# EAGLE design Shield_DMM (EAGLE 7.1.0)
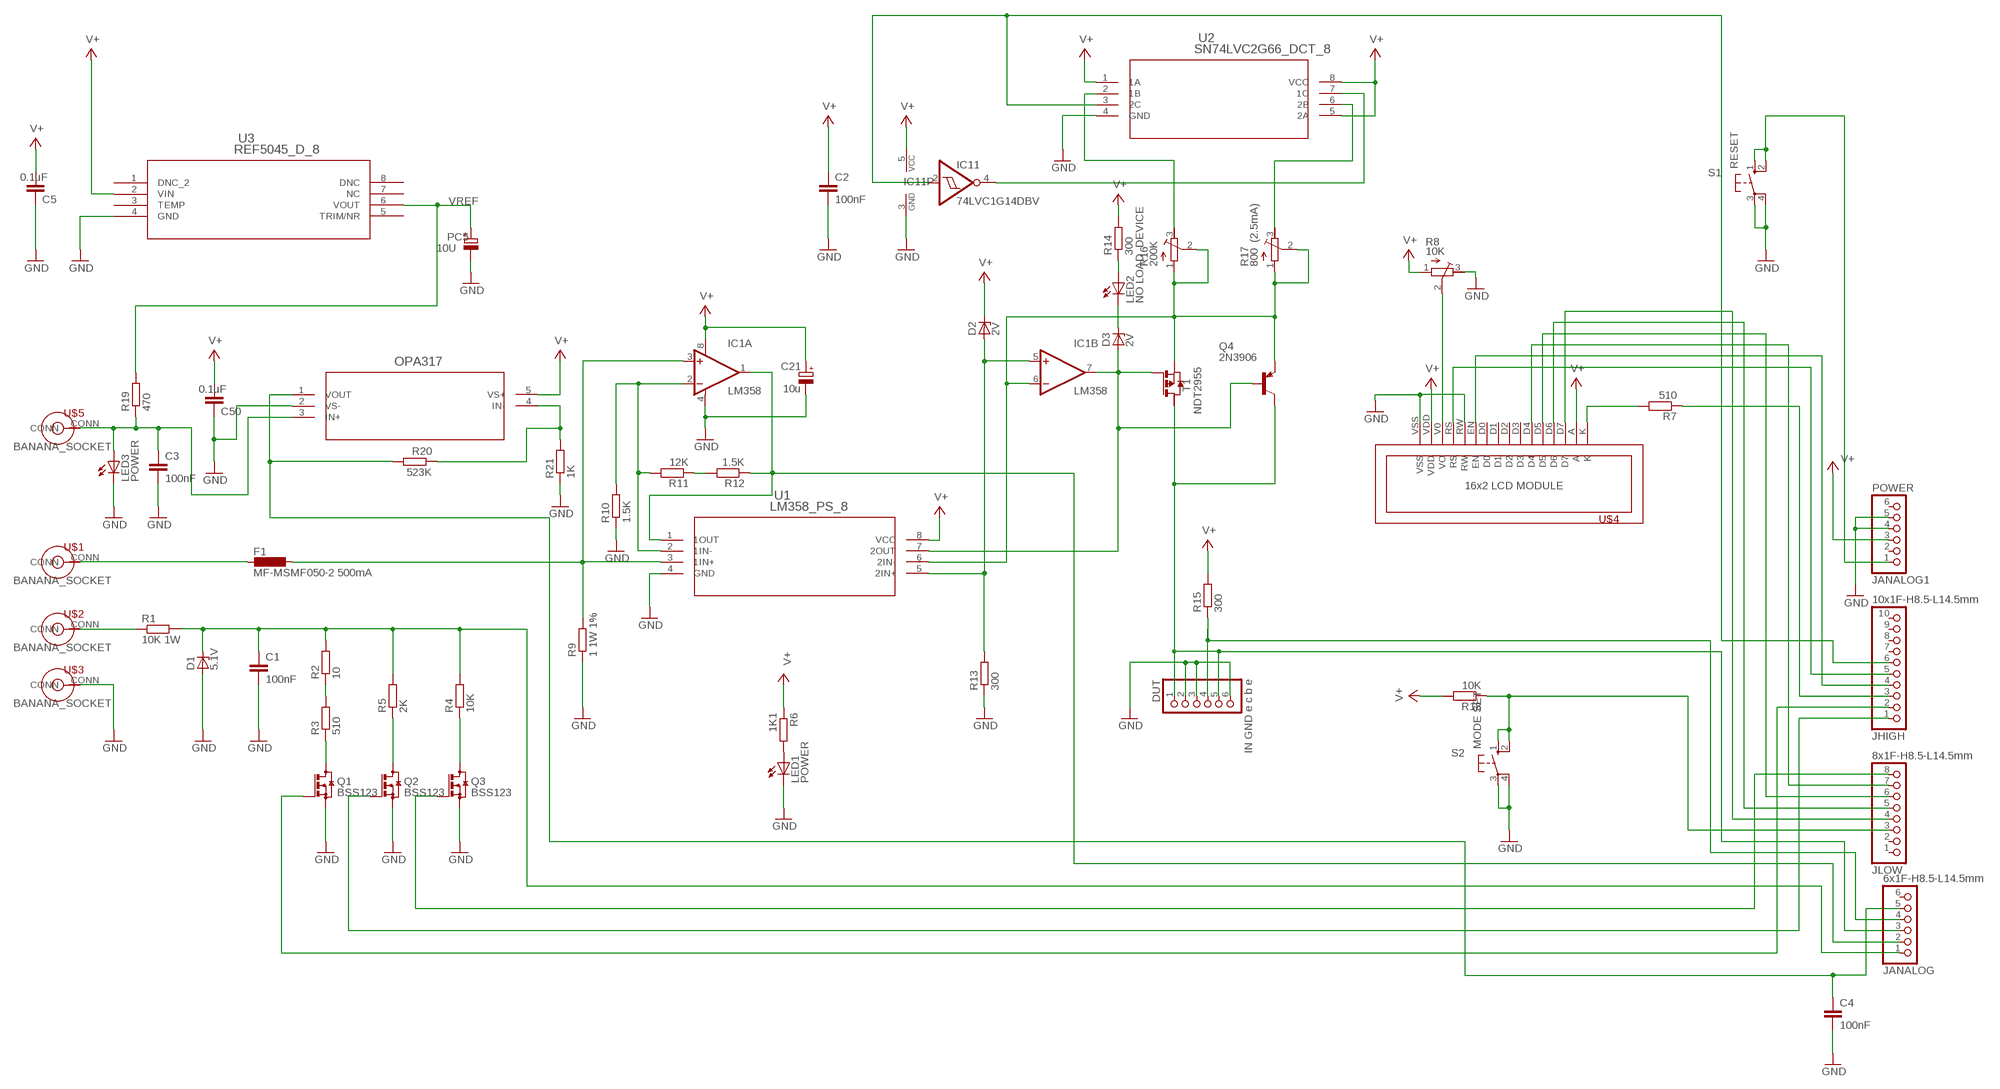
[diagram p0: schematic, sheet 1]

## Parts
C1  100nF  C-EUC0805  [C0805]
C2  100nF  C-EUC0805  [C0805]
C3  100nF  C-EUC0805  [C0805]
C4  100nF  C-EUC0805  [C0805]
C5  0.1uF  C-EUC0805  [C0805]
C21  10u  CPOL-EU085CS-1AR  [085CS_1AR]
C50  0.1uF  C-EUC0805  [C0805]
D1  5.1V  BZV10  [DO34Z7]
D2  2V  BZV10  [DO34Z7]
D3  2V  BZV10  [DO34Z7]
DUT  IN GND e c b e  PINHD-1X6  [1X06]
F1  MF-MSMF050-2 500mA  L-EUL1812  [L1812]
IC1  LM358  OPA2340U  [SO08]
IC11  74LVC1G14DBV  [SOT23-5]
JANALOG  6x1F-H8.5-L14.5mm  PINHD-1X6  [1X06]
JANALOG1  POWER  PINHD-1X6  [1X06]
JHIGH  10x1F-H8.5-L14.5mm  PINHD-1X10  [1X10]
JLOW  8x1F-H8.5-L14.5mm  PINHD-1X8  [1X08]
LED1  POWER  LEDCHIPLED_0805  [CHIPLED_0805]
LED2  NO LOAD DEVICE  LEDCHIPLED_0805  [CHIPLED_0805]
LED3  POWER  LEDCHIPLED_0805  [CHIPLED_0805]
OPA317  THS4281_DBV_5  [DBV5]
PC5  10U  CPOL-EUCT7343  [CT7343]
Q1  BSS123  [SOT23]
Q2  BSS123  [SOT23]
Q3  BSS123  [SOT23]
Q4  2N3906  [TO92]
R1  10K 1W  R-EU_0207/10  [0207/10]
R2  10  R-EU_R0805  [R0805]
R3  510  R-EU_R0805  [R0805]
R4  10K  R-EU_R0805  [R0805]
R5  2K  R-EU_R0805  [R0805]
R6  1K1  R-EU_R0805  [R0805]
R7  510  R-EU_R0805  [R0805]
R8  10K  R-TRIMM64W  [RTRIM64W]
R9  1 1W 1%  R-EU_0207/10  [0207/10]
R10  1.5K  R-EU_R0805  [R0805]
R11  12K  R-EU_R0805  [R0805]
R12  1.5K  R-EU_R0805  [R0805]
R13  300  R-EU_R0805  [R0805]
R14  300  R-EU_R0805  [R0805]
R15  300  R-EU_R0805  [R0805]
R16  200K  R-TRIMM64W  [RTRIM64W]
R17  800 (2.5mA)  R-TRIMM64W  [RTRIM64W]
R18  10K  R-EU_R0805  [R0805]
R19  470  R-EU_R0805  [R0805]
R20  523K  R-EU_R0603  [R0603]
R21  1K  R-EU_R0805  [R0805]
S1  RESET  10-XX  [B3F-10XX]
S2  MODE SET  10-XX  [B3F-10XX]
T1  NDT2955  PMOSSOT223  [SOT223]
U1  LM358_PS_8  [PS8]
U2  SN74LVC2G66_DCT_8  [DCT8]
U3  REF5045_D_8  REF5050_D_8  [D8]
U$1  BANANA_CONN  [BANANA_CONN]
U$2  BANANA_CONN  [BANANA_CONN]
U$3  Common  BANANA_CONN  [BANANA_CONN]
U$4  1602_LCM  [1602_LCM]
U$5  BANANA_CONN  [BANANA_CONN]

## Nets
GND: C1.2 C2.2 C3.2 C4.2 C5.2 C21.- C50.2 D1.A DUT.2 DUT.3 DUT.6 IC1.4(A:V-) IC11.3(GND) JANALOG1.4 JANALOG1.5 LED1.C LED3.C OPA317.2(VS-) PC5.- Q1.2(S) Q2.2(S) Q3.2(S) R8.3(E) R9.1 R10.1 R13.1 R21.1 S1.3(P) S1.4(P1) S2.3(P) S2.4(P1) U1.4(GND) U2.4(GND) U3.4(GND) U$3.CONN U$4.RW U$4.VSS
N$1: R1.1 U$2.CONN
N$2: C1.1 D1.C JANALOG.1 R1.2 R2.2 R4.2 R5.2
N$3: JHIGH.1 Q2.1(G)
N$4: Q3.3(D) R4.1
N$5: R2.1 R3.2
N$6: Q1.3(D) R3.1
N$7: JHIGH.2 Q1.1(G)
N$8: JLOW.8 Q3.1(G)
N$9: Q2.3(D) R5.1
N$10: LED1.A R6.2
N$11: R7.2 U$4.K
N$12: JHIGH.3 R7.1
N$13: R8.2(S) U$4.V0(VO)
N$14: JHIGH.4 U$4.EN
N$15: JHIGH.5 U$4.RS
N$16: JLOW.7 U$4.D4
N$17: JLOW.6 U$4.D5
N$18: JLOW.4 U$4.D7
N$19: JLOW.3 R18.1 S2.1(S) S2.2(S1)
N$20: F1.2 U$1.CONN
N$21: F1.1 IC1.3(A:+IN) R9.2 U1.3(1IN+)
N$22: IC1.2(A:-IN) R10.2 R11.2 U1.2(1IN-)
N$23: D2.A IC1.5(B:+IN) R13.2 U1.5(2IN+)
N$24: R11.1 R12.2
N$25: IC1.1(A:OUT) JANALOG.2 R12.1 U1.1(1OUT)
N$26: OPA317.4(IN-) R20.1 R21.2
N$27: IC1.6(B:-IN) Q4.3(E) R16.1(A) R16.2(S) R17.1(A) R17.2(S) T1.3(S) U1.6(2IN-)
N$28: D3.C LED2.C
N$29: LED2.A R14.1
N$30: DUT.1 DUT.5 JANALOG.3 Q4.1(C) T1.2(D)
N$31: JANALOG1.1 S1.1(S) S1.2(S1)
N$32: DUT.4 JANALOG.4 R15.1
N$33: JLOW.5 U$4.D6
N$34: IC11.2(I) JHIGH.6 U2.3(2C)
N$35: R16.3(E) U2.2(1B)
N$36: IC11.4(O) U2.7(1C)
N$38: D3.A IC1.7(B:OUT) Q4.2(B) T1.1(G) U1.7(2OUT)
N$39: R17.3(E) U2.6(2B)
V+: C2.1 C5.1 C21.+ C50.1 D2.C IC1.8(A:V+) IC11.5(VCC) JANALOG1.3 OPA317.5(VS+) R6.1 R8.1(A) R14.2 R15.2 R18.2 U1.8(VCC) U2.1(1A) U2.5(2A) U2.8(VCC) U3.2(VIN) U$4.A U$4.VDD
VR: C3.1 LED3.A OPA317.3(IN+) R19.1 U$5.CONN
VR1: C4.1 JANALOG.5 OPA317.1(VOUT) R20.2
VREF: PC5.+ R19.2 U3.6(VOUT)
Unconnected: JANALOG1.2 JANALOG1.6 JANALOG.6 JHIGH.7 JHIGH.8 JHIGH.9 JHIGH.10 JLOW.1 JLOW.2 T1.4(D2) U3.1(DNC_2) U3.3(TEMP) U3.5(TRIM/NR) U3.7(NC) U3.8(DNC) U$4.D0 U$4.D1 U$4.D2 U$4.D3

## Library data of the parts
C1-C5 C50 = rcl:C-EU: CAPACITOR, European symbol
C21 PC5 = rcl:CPOL-EU: POLARIZED CAPACITOR, European symbol
D1-D3 = diode:BZV10: Z DIODE
DUT JANALOG JANALOG1 = pinhead:PINHD-1X6: PIN HEADER
F1 = rcl:L-EU: INDUCTOR, European symbol
IC1 = burr-brown:OPA2340: Single-Supply, Rail-to-Rail Operational Amplifiers MicroAmplifier(TM) Series; Product Folder:OPA2340; MF: TEXAS INSTRUMENTS; MPN: OPA2340UA; OC_FARNELL: 1101541; OC_NEWARK: 36K7581
IC11 = 74xx-little-de:74*1G14: Single Schmitt-Trigger Inverter Gate
JHIGH = SmartPrj:PINHD-1X10: PIN HEADER
JLOW = SmartPrj:PINHD-1X8: PIN HEADER
LED1-LED3 = led:LED: LED
OPA317 = THS4281_DBV:THS4281_DBV_5; DATASHEETURL: http://www.ti.com/lit/gpn/THS4281; DESCRIPTION: Very Low-Power High Speed Rail-To-Rail Input/Output Voltage Feedback Operational Amplifier; FAMILY_NAME: RAIL TO RAIL; GENERIC_PART_NUMBER: THS4281; INDUSTRY_STD_PKG_TYPE: SOT-23; MANUFACTURER: Texas Instruments; MANUFACTURER_PART_NUMBER: ths4281_dbv_5; PACKAGE_DESIGNATOR: DBV; PIN_COUNT: 5; VENDOR: Texas Instruments
Q1-Q3 = transistor-small-signal:BSS123: N-CHANNEL MOS FET
Q4 = transistor-pnp:2N3906: PNP Transistor
R1-R7 R9-R15 R18-R21 = rcl:R-EU_: RESISTOR, European symbol
R8 R16 R17 = rcl:R-TRIMM: Trimm resistor
S1 S2 = switch-omron:10-XX: OMRON SWITCH
T1 = zetex:PMOSSOT223: MOS FET
U1 = LM358PS:LM358_PS_8; DATASHEETURL: http://www.ti.com/lit/gpn/LM358; DESCRIPTION: Dual Operational Amplifiers; FAMILY_NAME: STANDARD LINEAR AMPLIFIER; GENERIC_PART_NUMBER: LM358; INDUSTRY_STD_PKG_TYPE: SO; MANUFACTURER: Texas Instruments; PACKAGE_DESIGNATOR: PS; PIN_COUNT: 8
U2 = SN74LVC2G66_DCT_8:SN74LVC2G66_DCT_8; DATASHEETURL: http://www.ti.com/lit/gpn/SN74LVC2G66; DESCRIPTION: Dual Analog Switch; FAMILY_NAME: ANALOG SWITCH/MULTIPLEXER(less than or equal to 5V); GENERIC_PART_NUMBER: SN74LVC2G66; INDUSTRY_STD_PKG_TYPE: SM8; MANUFACTURER: Texas Instruments; MANUFACTURER_PART_NUMBER: sn74lvc2g66_dct_8; PACKAGE_DESIGNATOR: DCT; PIN_COUNT: 8; VENDOR: Texas Instruments
U3 = REF5050:REF5050_D_8; DATASHEETURL: http://www.ti.com/lit/gpn/REF5050; DESCRIPTION: Low Noise, Very Low Drift, Precision VOLTAGE REFERENCE; FAMILY_NAME: SERIES VOLTAGE REFERENCE; GENERIC_PART_NUMBER: REF5050; INDUSTRY_STD_PKG_TYPE: SOIC; MANUFACTURER: Texas Instruments; MANUFACTURER_PART_NUMBER: ref5050_d_8; PACKAGE_DESIGNATOR: D; PIN_COUNT: 8; VENDOR: Texas Instruments
U$1-U$3 U$5 = banana-socket:BANANA_CONN: BANANA SOCKET 3.5 mm.
U$4 = 1602-LCM:1602_LCM

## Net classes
0 default: width 0.152 mm, drill 0.61 mm, clearance 0.152 mm
1 power: width 0.152 mm, drill 0.61 mm, clearance 0.152 mm
2 VIN: width 0.305 mm, drill 0.61 mm, clearance 0.152 mm
3 usbvcc: width 0.508 mm, drill 0.61 mm, clearance 0.254 mm

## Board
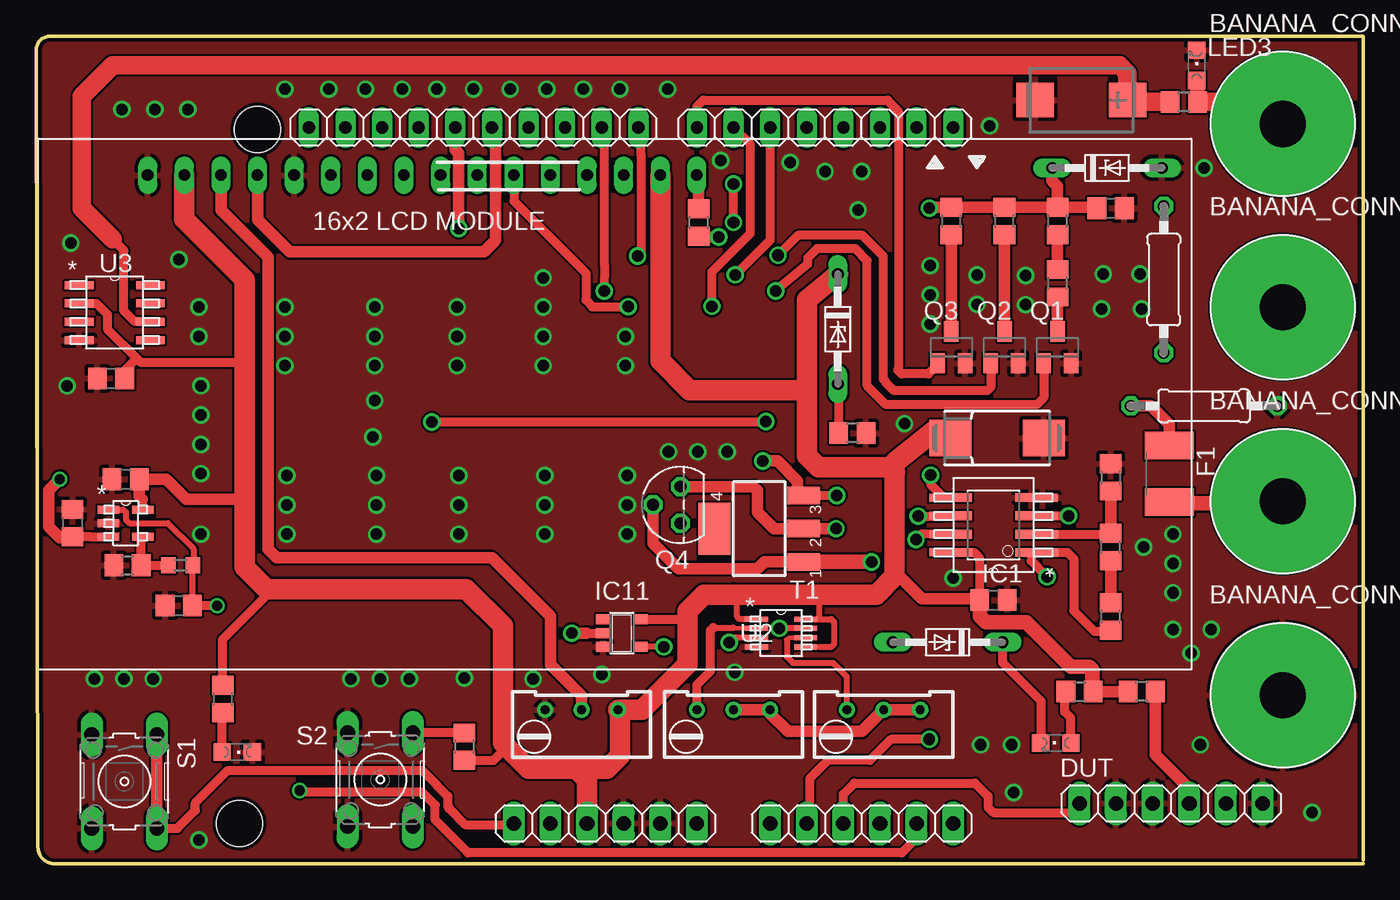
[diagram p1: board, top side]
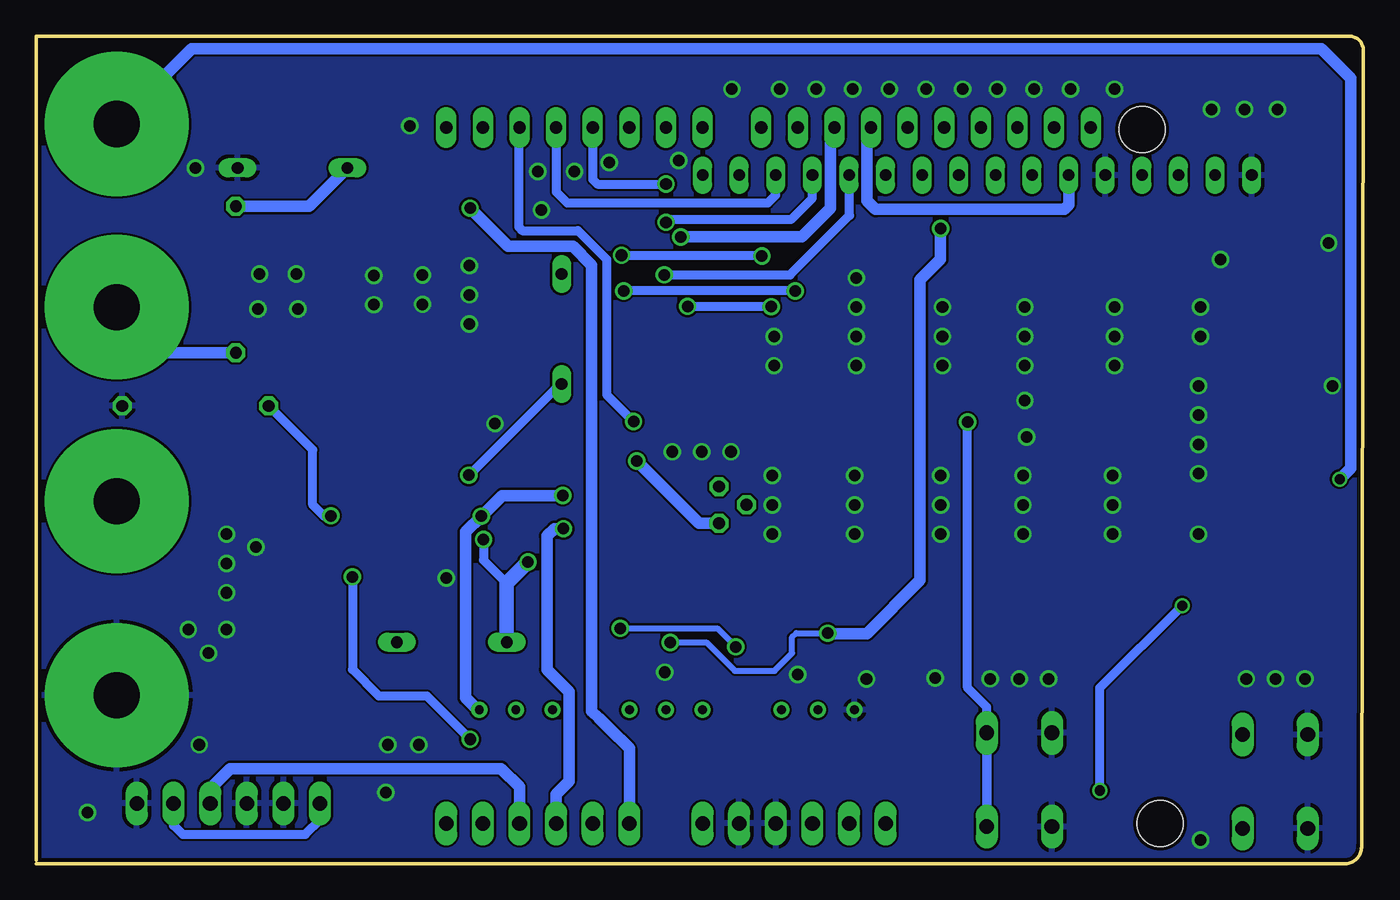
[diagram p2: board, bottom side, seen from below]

Size 92.09 x 57.4 mm. Coordinates in mm from the lower left corner, seen from the top.
Outline: 92.07,0.24 92.07,57.4 1,57.4 arc90 0,56.4 0.13,1.25 arc90 1.25,0 92.09,0
Copper layers (1*16): Top 0.035mm / dielectric 1.5mm / Bottom 0.035mm
Design rules "ITEADstudio_DRC": minimum track width 6mil, minimum drill 12mil, track to track 6mil, track to pad 6mil, pad to pad 6mil, via to via 6mil, smd to smd 0mil, copper to edge 10mil, drill to drill 10mil, minimum pad ring 10mil, minimum via ring 6mil, stop-mask expansion 2mil, vias tented up to drill 100mil, thermal gap 10mil
Holes 3.2 mm at 15.37,50.93 14.1,2.79

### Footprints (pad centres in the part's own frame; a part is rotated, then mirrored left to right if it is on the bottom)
C0805 = smd 1.3 x 1.5: 1 -0.95,0; 2 0.95,0
085CS_1AR = smd 2.9 x 2.5: + 3.25,0; - -3.25,0
DO34Z7 = drill 0.813 long: A 3.81,0; C -3.81,0
1X06 = drill 1.016 long: 1 -6.35,0; 2 -3.81,0; 3 -1.27,0; 4 1.27,0; 5 3.81,0; 6 6.35,0
L1812 = smd 1.9 x 3.4: 1 -1.95,0; 2 1.95,0
SO08 = smd 0.61 x 2.21: 1 -1.905,-2.616; 2 -0.635,-2.616; 3 0.635,-2.616; 4 1.905,-2.616; 5 1.905,2.616; 6 0.635,2.616; 7 -0.635,2.616; 8 -1.905,2.616
SOT23-5 = smd 0.69 x 0.99: 1 -0.95,-1.29; 2 0,-1.29; 3 0.95,-1.29; 4 0.95,1.3; 5 -0.95,1.3
1X10 = drill 0.85 pad 1.422 long: 1 -11.43,0; 2 -8.89,0; 3 -6.35,0; 4 -3.81,0; 5 -1.27,0; 6 1.27,0; 7 3.81,0; 8 6.35,0; 9 8.89,0; 10 11.43,0
1X08 = drill 0.85 pad 1.422 long: 1 -8.89,0; 2 -6.35,0; 3 -3.81,0; 4 -1.27,0; 5 1.27,0; 6 3.81,0; 7 6.35,0; 8 8.89,0
CHIPLED_0805 = smd 1.2 x 1.2: A 0,-1.05; C 0,1.05
DBV5 = smd 1.473 x 0.559: 1 -1.194,0.94; 2 -1.194,0; 3 -1.194,-0.94; 4 1.194,-0.94; 5 1.194,0.94
CT7343 = smd 2.6 x 2.4: + -3.2,0; - 3.2,0
SOT23 = smd 1 x 1.4: 1 -0.95,-1.1; 2 0.95,-1.1; 3 0,1.1
TO92 = drill 0.813 octagon: 1 1.27,0; 2 0,1.905; 3 -1.27,0
0207/10 = drill 0.813 octagon: 1 -5.08,0; 2 5.08,0
R0805 = smd 1.3 x 1.5: 1 -0.95,0; 2 0.95,0
RTRIM64W = drill 0.61: 1 1.27,-2.54; 2 1.27,0; 3 1.27,2.54
R0603 = smd 1 x 1.1: 1 -0.85,0; 2 0.85,0
B3F-10XX = drill 1.016 long: 1 -3.251,2.261; 2 3.251,2.261; 3 -3.251,-2.261; 4 3.251,-2.261
SOT223 = smd 1.219 x 2.235: 1 -2.311,-3.099; 2 0,-3.099; 3 2.311,-3.099 | smd 3.6 x 2.2: 4 0,3.099
PS8 = smd 2.057 x 0.559: 1 -3.429,1.905; 2 -3.429,0.635; 3 -3.429,-0.635; 4 -3.429,-1.905; 5 3.429,-1.905; 6 3.429,-0.635; 7 3.429,0.635; 8 3.429,1.905
DCT8 = smd 1.575 x 0.356: 1 -1.702,0.965; 2 -1.702,0.33; 3 -1.702,-0.33; 4 -1.702,-0.965; 5 1.702,-0.965; 6 1.702,-0.33; 7 1.702,0.33; 8 1.702,0.965
D8 = smd 1.981 x 0.559: 1 -2.464,1.905; 2 -2.464,0.635; 3 -2.464,-0.635; 4 -2.464,-1.905; 5 2.464,-1.905; 6 2.464,-0.635; 7 2.464,0.635; 8 2.464,1.905
BANANA_CONN = drill 3.2 pad 10: CONN 0,0
1602_LCM = drill 0.8 long: A 43.18,34.29; D0 22.86,34.29; D1 25.4,34.29; D2 27.94,34.29; D3 30.48,34.29; D4 33.02,34.29; D5 35.56,34.29; D6 38.1,34.29; D7 40.64,34.29; EN 20.32,34.29; K 45.72,34.29; RS 15.24,34.29; RW 17.78,34.29; V0 12.7,34.29; VDD 10.16,34.29; VSS 7.62,34.29

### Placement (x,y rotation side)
C1  74.55,45.47 0 top
C2  66.42,18.29 0 top
C3  2.54,23.62 90 top
C4  9.91,17.91 180 top
C5  5.21,33.66 180 top
C21  66.67,29.53 180 top
C50  6.22,26.67 180 top
D1  74.3,48.26 0 top
D2  55.63,37.08 270 top
D3  63.25,15.37 180 top
DUT  78.74,4.19 0 top
F1  78.61,27.05 270 top
IC1  66.42,23.5 90 top
IC11  40.64,16 270 top
JANALOG  57.28,2.79 0 top
JANALOG1  39.5,2.79 0 top
JHIGH  30.35,51.05 180 top
JLOW  54.74,51.05 180 top
LED1  13.97,7.75 270 top
LED2  70.74,8.38 90 top
LED3  80.52,55.37 0 top
OPA317  6.22,23.62 0 top
PC5  72.52,52.96 180 top
Q1  70.87,35.81 0 top
Q2  67.18,35.81 0 top
Q3  63.5,35.81 0 top
Q4  44.7,24.89 90 top
R1  78.23,40.51 90 top
R2  70.87,44.58 90 top
R3  70.87,40.26 90 top
R4  63.5,44.58 90 top
R5  67.18,44.58 90 top
R6  12.95,11.43 270 top
R7  45.97,44.48 90 top
R8  37.85,9.4 90 top
R9  81.03,31.75 180 top
R10  74.55,26.8 270 top
R11  74.55,21.97 90 top
R12  74.55,17.14 90 top
R13  56.64,29.87 180 top
R14  72.39,11.94 0 top
R15  76.71,11.94 180 top
R16  48.39,9.4 90 top
R17  58.8,9.4 90 top
R18  29.72,8.13 270 top
R19  79.63,52.83 180 top
R20  10.03,20.7 0 top
R21  6.35,20.7 0 top
S1  6.13,5.7 270 top
S2  23.88,5.83 270 top
T1  50.16,23.24 90 top
U1  66.42,23.5 180 top
U2  51.69,16 0 top
U3  5.46,38.23 0 top
U$1  86.49,25.15 0 top
U$2  86.49,38.61 0 top
U$3  86.49,11.68 0 top
U$4  0.13,13.46 0 top
U$5  86.49,51.31 0 top

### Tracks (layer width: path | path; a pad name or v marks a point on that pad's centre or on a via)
GND  (via drill 0.8)
  Top 0.305: IC1.4 U1.4
  other vias: 76.58,40.89 76.71,38.48 73.91,38.48 74.04,40.89 62.04,39.46 62.03,37.44 62.03,41.48 40.89,36.58 40.89,34.54 35.18,40.64 41.02,24.89 41.02,22.86 41.02,26.92 35.18,36.58 35.18,34.54 35.18,38.61 35.31,24.89 35.31,22.86 35.31,26.92 29.21,36.58 29.21,34.54 29.21,38.61 29.34,24.89 29.34,22.86 29.34,26.92 23.49,36.58 23.49,34.54 23.49,38.61 23.62,24.89 23.62,22.86 23.62,26.92 17.27,36.58 17.27,34.54 17.27,38.61 17.4,24.89 17.4,22.86 17.4,26.92 11.3,36.58 11.43,33.15 11.3,38.61 11.43,31.12 11.43,22.86 11.43,27.05 2.41,43.05 2.16,33.15 9.91,41.91 23.37,29.59 11.43,29.08 23.49,32.13 65.53,8.25 67.82,4.95 67.69,8.25 76.83,21.97 78.87,18.8 78.87,22.86 80.77,8.25 88.52,3.56 78.87,16.26 80.14,14.61 81.53,16.26 78.87,20.83 45.91,28.58 43.88,28.58 47.94,28.58 6.1,12.83 8.13,12.83 4.06,12.83 23.88,12.83 25.91,12.83 21.84,12.83 48.48,13.28 39.24,13.13 68.64,38.77 68.64,40.81 65.28,38.8 65.28,40.83 29.72,12.88 34.48,12.81 60.25,30.52 54.74,48.01 52.32,48.64 47.5,48.77 57.02,45.34 57.28,48.01 11.3,1.65 63.63,19.81 66.17,51.18 81.03,48.26 5.97,52.32 8.26,52.32 10.54,52.32 17.27,53.72 20.32,53.72 22.86,53.72 25.4,53.72 27.81,53.72 30.35,53.72 32.89,53.72 35.43,53.72 37.97,53.72 40.51,53.72 43.82,53.72
  pour Bottom: -1.4,60.2 93.85,60.2 94.11,-1.02 -1.14,-1.02
  pour Top: -2.67,60.96 95.12,60.96 95.38,-2.29 -2.41,-2.29
N$1
  Bottom 0.813: R1.1 83.82,35.43 U$2.CONN
N$2  (via drill 0.8)
  Top 0.813: D1.C 70.48,47.37 70.87,46.99 R2.2 | R2.2 73.54,45.53 C1.1 | R2.2 R5.2 R4.2 62.04,45.53 v61.98,45.47
  Bottom 0.813: JANALOG.1 50.93,8 52.32,9.4 52.34,9.4 53.06,10.12 53.07,10.12 53.54,10.59 53.54,41.52 54.85,42.82 59.33,42.82 v61.98,45.47 | R1.2 73.15,45.59 D1.C
N$3  (via drill 0.8)
  Top 0.61: Q2.1 66.23,33.06 65.99,32.82 59.53,32.82 58.9,33.44 58.9,33.49 58.79,33.6 58.79,42.13 57.34,43.57 52.85,43.57 v51.47,42.2 | JHIGH.1 41.95,50.75 41.95,49.2 41.99,49.16 41.99,42.41 v41.73,42.15
  Bottom 0.61: 41.9,42.19 v41.73,42.15 41.89,42.19 51.26,42.19 v51.47,42.2
N$4
  Top 0.813: R4.1 Q3.3
N$5
  Top 0.813: R2.1 R3.2
N$6
  Top 0.813: R3.1 Q1.3
N$7  (via drill 0.8)
  Top 0.61: Q1.1 69.92,32.34 69.43,31.85 58.97,31.85 57.66,33.16 57.66,41.83 56.82,42.67 54.2,42.67 53.54,42.01 53.54,41.6 v51.31,39.73 | JHIGH.2 39.43,50.86 39.43,41.57 v39.42,39.73
  Bottom 0.61: v39.42,39.73 v51.31,39.73
N$8
  Top 0.61: Q3.1 62.55,34.6 61.93,33.97 60.05,33.97 59.78,34.24 59.82,34.28 59.82,52.2 59.07,52.96 46.28,52.96 45.85,52.53 JLOW.8
N$9
  Top 0.813: R5.1 Q2.3
N$10
  Top 0.61: LED1.A 12.92,10.45 R6.2
N$11
  Top 0.813: R7.2 45.97,47.62 U$4.K
N$12  (via drill 0.8)
  Top 0.813: R7.1 47.32,43.46 v47.37,43.47
  Bottom 0.813: v47.37,43.47 38.94,43.47 36.97,45.47 36.97,50.79 JHIGH.3
N$13
  Top 0.813: R8.2 37.85,11.65 35.69,13.8 35.69,17.16 31.64,21.21 16.69,21.21 16.09,21.81 16.09,42.05 12.83,45.31 U$4.V0
N$14
  Bottom 0.813: U$4.EN 20.45,45.7 20.76,45.38 33.85,45.38 34.44,45.97 34.44,50.77 JHIGH.4
N$15
  Top 0.813: U$4.RS 15.37,44.68 17.6,42.44 31.09,42.44 31.89,43.26 31.88,50.69 JHIGH.5
N$16  (via drill 0.8)
  Top 0.61: U$4.D4 33.15,45.96 38.15,40.96 38.15,39.12 38.6,38.62 v41.09,38.63 | v46.89,38.66 46.89,41.05 49.55,43.71 49.55,49.89 JLOW.7
  Bottom 0.61: v41.09,38.63 46.86,38.63 v46.89,38.66
N$17  (via drill 0.8)
  Top 0.61: JLOW.6 50.93,43.26 v48.51,40.84
  Bottom 0.61: v48.51,40.84 39.78,40.84 35.65,44.97 35.65,47.71 U$4.D5
N$18
  Bottom 0.61: JLOW.4 56.01,46.6 55.25,45.83 41.33,45.83 40.78,46.38 40.78,47.74 U$4.D7
N$19  (via drill 0.8)
  Top 0.61: R18.1 S2.1 | v27.46,30.64 50.61,30.64 v50.64,30.67
  Bottom 0.61: S2.1 S2.2 26.14,10.87 27.47,12.21 27.47,30.63 v27.46,30.64 | JLOW.3 58.6,51 58.6,44.14 58.36,43.9 54.5,43.9 52.5,41.91 52.5,32.54 v50.64,30.67
N$20
  Top 1.016: F1.2 78.69,25.02 86.36,25.02 U$1.CONN
N$21  (via drill 0.8)
  Top 0.61: IC1.3 U1.3 v71.63,24.13
  Top 0.813: F1.1 78.61,30.48 77.34,31.75 R9.2
  Bottom 0.61: v71.63,24.13 72.14,24.13 72.9,24.89 72.9,28.7 R9.2
N$22
  Top 0.305: IC1.2 U1.2
  Top 0.61: U1.2 74.49,22.86 R11.2
  Top 0.813: R11.2 R10.2
N$23  (via drill 0.8)
  Top 0.305: IC1.5 U1.5
  Top 0.61: v62.07,26.95 62.07,26.33 U1.5 | R13.2 55.69,33.21 D2.A
  Bottom 0.61: D2.A 55.78,33.27 55.78,33.24 v62.07,26.95
N$24
  Top 0.813: R12.2 R11.1
N$25  (via drill 0.8)
  Top 0.305: IC1.1 U1.1
  Top 0.61: U1.1 71.55,21.59 71.98,21.16 71.98,17.56 73.43,16.12 74.47,16.12 R12.1 | IC1.1 69.04,21.01 v70.14,19.9 | v61.98,8.64 59.32,8.64 57.85,7.16 54.93,7.16 53.66,5.89 53.66,2.98 JANALOG.2
  Bottom 0.61: v70.14,19.9 70.14,13.47 68.31,11.65 64.99,11.65 v61.98,8.64
N$26
  Top 0.61: OPA317.4 7.3,22.57 R21.2 R20.1
N$27  (via drill 0.8)
  Top 0.305: IC1.6 U1.6
  Top 0.61: T1.3 55.52,25.55 v55.54,25.54 | v61.19,24.11 62.97,24.11 U1.6
  Top 0.813: R16.2 R16.1 50.93,10.41 52.16,9.18 57.31,9.18 R17.2 R17.1 | v50.42,27.94 51.44,27.94 52.83,26.54 52.83,25.98 T1.3
  Bottom 0.813: R17.1 61.46,10.67 62.29,11.51 62.29,23.01 v61.19,24.11 59.75,25.54 v55.54,25.54 | Q4.3 46.1,23.62 v50.42,27.94
N$28
  Top 0.61: D3.C 67.06,13.97 69.72,11.3 69.72,8.42 LED2.C
N$29
  Top 0.61: LED2.A 71.79,10.13 71.37,10.54 71.37,11.87 R14.1
N$30  (via drill 0.8)
  Top 0.61: JANALOG.3 56.01,4.83 56.77,5.59 65.15,5.59 66.04,4.7 66.04,3.94 66.42,3.56 71.75,3.56 DUT.1
  Top 0.813: v55.5,23.24 T1.2 51.18,23.24 50.04,24.38 50.04,25.91 49.78,26.16 Q4.1
  Bottom 0.61: DUT.5 82.55,2.67 81.91,2.03 73.41,2.03 72.39,3.05 DUT.1
  Bottom 0.813: v55.5,23.24 56.13,23.24 56.64,22.73 56.64,13.46 55.12,11.94 55.12,5.71 56.01,4.83 JANALOG.3
N$31
  Top 0.61: S1.2 9.81,2.45 11.05,3.7 11.05,4.22 13.31,6.48 26.77,6.48 27.85,5.4 27.93,5.32 28.56,4.69 28.56,4 28.64,3.92 28.64,3.85 29.77,2.72 33.07,2.72 JANALOG1.1
  Top 0.813: S1.1 S1.2
N$32
  Top 0.813: DUT.4 80.01,5.21 77.66,7.56 R15.1
  Bottom 0.813: JANALOG.4 58.55,5.33 59.82,6.6 78.61,6.6 80.01,5.21 DUT.4
N$33  (via drill 0.8)
  Top 0.61: v48.39,44.49 v48.39,47.14
  Bottom 0.61: JLOW.5 53.47,47.46 53.15,47.14 v48.39,47.14 | U$4.D6 38.24,47.74 38.24,46.16 39.73,44.68 48.2,44.68 v48.39,44.49
N$34  (via drill 0.8)
  Top 0.406: U2.3 48.4,15.67 v48.08,15.35
  Top 0.61: 38.19,15.99 39.34,15.99 IC11.2
  Top 0.813: JHIGH.6 29.08,49.5 29.3,49.29 29.3,44.09 v29.34,44.06 | v37.16,15.99 38.18,15.98 38.19,15.99
  Bottom 0.406: v48.08,15.35 45.58,15.35 43.61,13.39 40.86,13.39 39.64,14.61 39.64,15.71 IC11.2 37.17,16 v37.16,15.99
  Bottom 0.813: v29.34,44.06 29.34,41.91 30.76,40.49 30.76,19.65 34.44,15.96 36.69,15.96 v37.16,15.99
N$35
  Top 0.305: 48.4,16.35 49.4,16.35 49.44,16.31 49.96,16.31 U2.2
  Top 0.406: 46.99,16.38 48.36,16.38 48.4,16.35
  Top 0.61: R16.3 45.85,12.41 46.77,13.33 46.77,16.17 46.99,16.38
N$36  (via drill 0.8)
  Top 0.406: U2.7 v51.56,16.33 | v43.55,15.05 IC11.4
  Bottom 0.406: v51.56,16.33 44.83,16.33 v43.55,15.05
N$38  (via drill 0.8)
  Top 0.305: U1.7 IC1.7
  Top 0.61: U1.7 61.44,22.87 v61.05,22.48
  Top 0.813: T1.1 50.52,20.93 50.04,20.45 44.58,20.45 42.8,22.23 Q4.2
  Top 1.016: v57.96,20.93 T1.1
  Bottom 0.61: v61.05,22.48 61.05,21.06 59.44,19.46
  Bottom 1.016: D3.A 59.44,19.46 v57.96,20.93
N$39
  Top 0.305: U2.6 52.23,15.67 52.08,15.52
  Top 0.406: 52.08,15.52 52.08,14.35 52.5,13.93 55.3,13.93 56.22,13 56.22,10.71 R17.3
V+
  Top 0.305: 54.33,15.02 53.4,15.02 U2.5 | U2.8 54.3,16.97 54.34,17.01 | 62.34,30.07 62.29,29.86 59.58,27.14
  Top 0.406: U2.1 48.82,16.97 48.64,17.14 48.64,18.42 48.39,18.67 | U2.8 55.17,16.97 55.37,16.76 55.37,15.24 55.19,15.06 55.18,15.06 55.14,15.02 54.33,15.02 | 54.34,17.01 54.34,18.39 54.06,18.67
  Top 0.61: IC11.5 45.02,16.95 45.21,17.14 | U1.8 IC1.8 65.09,21.59 65.44,21.23 65.44,18.32 C2.1 | R18.2 31.73,7.18 32.66,8.11 | R6.1 12.95,15.58 16.42,19.05 | U3.2 4.19,38.86 4.95,38.1 4.95,37.08 6.98,35.05 | 6.98,35.05 7.24,34.8 14.35,34.8 14.48,34.67 | C5.1 6.16,34.22 6.98,35.05 | 7.37,25.27 7.37,24.61 OPA317.5
  Top 0.813: 59.56,19.94 59.89,19.94 61.44,18.39 65.37,18.39 C2.1 | R14.2 R15.2 | 7.37,25.27 7.17,25.47 C50.1 9.02,26.67 10.41,25.27 14.35,25.27 14.48,25.15
  Top 1.016: C2.1 65.47,17.18 65.91,16.74 68.69,16.74 71.78,13.65 73.09,13.65 73.28,13.46 73.28,12 R14.2
  Top 1.422: C21.+ 62.74,30.1 62.34,30.07 59.56,27.81 59.56,19.94 58.29,18.67 54.06,18.67 48.39,18.67 46.36,18.67 45.21,17.53 45.21,17.14 45.21,13.84 42.04,10.67 R8.1 40.51,10.55 40.51,7.49 39.62,6.6 37.47,6.6 | D2.C 53.48,39.13 53.48,32.6 | JANALOG1.3 38.23,5.84 37.47,6.6 | 37.47,6.6 34.16,6.6 32.66,8.11 32.39,8.38 32.39,16.51 29.84,19.05 16.42,19.05 16,19.05 14.48,20.57 14.48,25.15 14.48,34.67 14.48,40.51 10.29,44.7 U$4.VDD | 59.58,27.14 59.58,27.15 59.23,27.5 54.27,27.5 53.48,28.28 53.48,32.6 | U$4.A 43.31,34.89 45.34,32.85 53.23,32.85 53.48,32.6
VR  (via drill 0.7)
  Top 0.406: OPA317.3 2.41,22.68 2.41,22.61
  Top 0.61: C3.1 3.69,22.68 OPA317.3
  Top 0.813: 2.41,22.61 1.65,22.61 0.89,23.37 0.89,25.91 v1.65,26.67
  Top 1.016: LED3.A 80.58,54.32 R19.1
  Top 1.27: R19.1 84.96,52.83 U$5.CONN
  Bottom 0.813: U$5.CONN 81.28,56.52 2.92,56.52 0.89,54.48 0.89,27.43 v1.65,26.67
VR1  (via drill 0.7)
  Top 0.406: OPA317.1 6.04,24.56 6.22,24.38 6.22,23.88 6.48,23.62 9.14,23.62 10.92,21.84 10.92,20.74 R20.2 10.86,20.67 C4.1
  Top 0.61: 61.09,1.78 60.07,0.76 29.97,0.76 27.69,3.05 27.69,4.06 26.8,4.95 18.41,4.95 v18.29,5.08 | v12.57,17.91 C4.1
  Top 0.813: 61.09,1.78 JANALOG.5
  Bottom 0.61: v18.29,5.08 18.29,12.19 v12.57,17.91
VREF
  Top 0.61: U3.6 6.86,37.59 6.1,38.35 6.1,42.54 5.33,43.31
  Top 1.27: R19.2 76.45,52.83 76.33,52.96 PC5.+ 75.72,54.84 75.18,55.37 5.33,55.37 3.17,53.21 3.17,45.47 5.33,43.31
